(*此PLC项目为FB_XmlSrvWriteByName对应例程,FB_XmlSrvReadByName请打开名称为CX2020 XmlReadByName的PLC项目*)
PROGRAM MAIN
VAR
	ST_XmlWrite2: ST_XmlTest2;
	FB_XmlWriteByName: FB_XmlSrvWriteByName;
	b_Execute: BOOL;
	sSymName: T_MaxString :='MAIN.ST_XmlWrite2';		//要写入XML文件的PLC变量的名称
	sFilePath: T_MaxString:='C:\temp\Test.xml';			//Win7和Win10的系统路径和WinCE系统有一定区别，需要注意路径是否填写正确
	sXPath: T_MaxString:='/dataentry/MAIN.ST_XmlWrite2';
END_VAR

FB_XmlWriteByName(
	sNetId:= , 
	ePath:= PATH_GENERIC, 
	nMode:= XMLSRV_ADDMISSING, 
	sSymName:= sSymName, 
	sFilePath:= sFilePath, 
	sXPath:= sXPath, 
	bExecute:= b_Execute, 
	tTimeout:= , 
	bBusy=> , 
	bError=> , 
	nErrId=> );

END_PROGRAM
